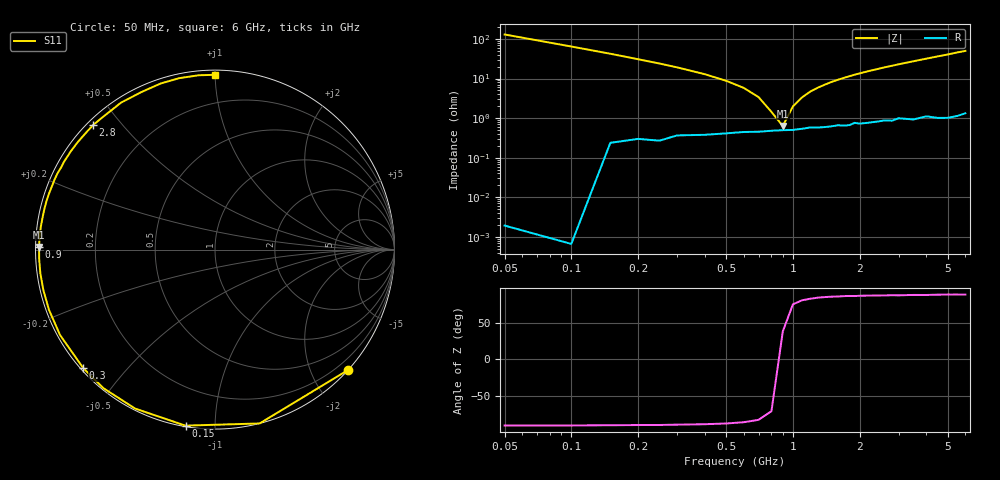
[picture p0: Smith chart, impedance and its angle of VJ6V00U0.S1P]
! Infineon Technologies  Discrete & RF Semiconductors
! BB 914
! Si Tuning Diode in SOT23
! VR = 6 V
! S-Parameters:  July  1999
# GHz  S  MA  R  50
!  f  S11
! GHz  MAG  ANG
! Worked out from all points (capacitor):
!   34 points, 50 MHz to 6 GHz, reference 50 ohm
!   read as one part to ground: C = 24.4 pF near 50 MHz
!   lowest |Z| = 633 mohm at 900 MHz (marker M1)
!   series resonance near 877.5 MHz, so ESL is about 1.3 nH
!   S11 on the Smith chart (normalised r, x): 50 MHz: 0.00, -2.60; 150 MHz: 0.00, -0.85; 300 MHz: 0.01, -0.38; 900 MHz: 0.01, +0.01; 2.8 GHz: 0.02, +0.42; 6 GHz: 0.03, +1.00
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0.05  1 -42.1
0.1  1 -75.6
0.15  0.9945 -99.5
0.2  0.9914 -116.7
0.25  0.9913 -128.8
0.3  0.9873 -138.0
0.4  0.9859 -151.1
0.5  0.9841 -160.1
0.6  0.9825 -166.8
0.7  0.9821 -172.3
0.8  0.981 -176.9
0.9  0.9803 179.1
1  0.9801 175.6
1.2  0.9771 169.3
1.5  0.976 161.2
1.6  0.9747 158.8
2  0.9733 149.8
2.2  0.9723 145.6
2.4  0.9711 141.8
2.6  0.9698 137.8
2.8  0.9711 134.4
3  0.9677 130.7
3.5  0.9719 122.6
4  0.9688 115.0
4.5  0.9737 108.0
5  0.9757 101.8
5.5  0.9756 95.3
6  0.9737 90.0
